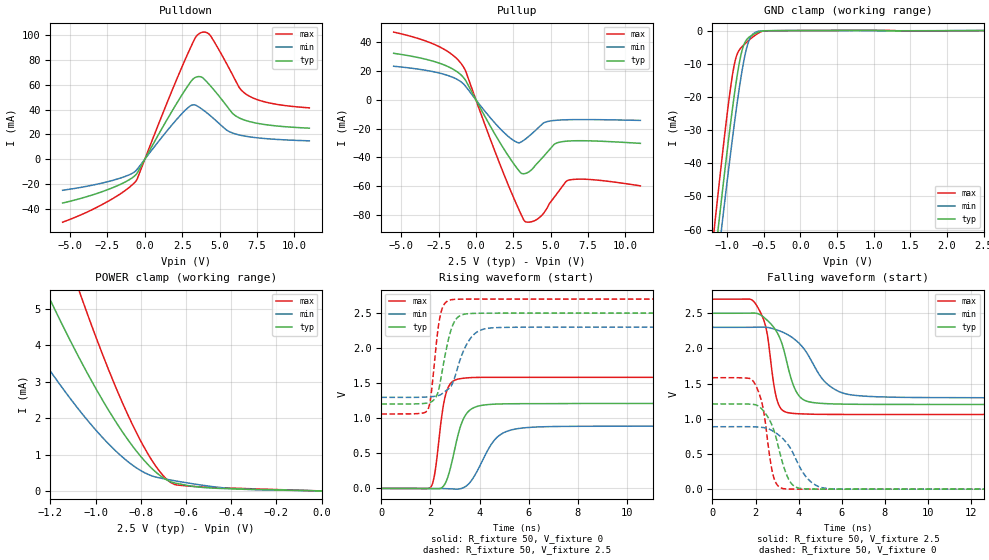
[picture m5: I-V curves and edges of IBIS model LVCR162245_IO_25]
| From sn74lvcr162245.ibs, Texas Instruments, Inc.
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[Model]   LVCR162245_IO_25
Model_type  I/O
Vinl=0.8
Vinh=2.0
Enable   Active-Low
Vref =   0
Rref =   500
Cref =   30p
Vmeas =   1.5
| variable   typ   min   max
C_comp   7.42pF   6.47pF   8.78pF
| C_pullup   5.98pF   4.73pF   8.31pF
| C_pulldown   5.48pF   4.75pF   6.82pF
| C_tri-state   7.42pF   6.47pF   8.78pF
[Temperature Range]   40   100   -40
| Ambient temperature   25   85   -40
[Voltage range]   2.5   2.3   2.7
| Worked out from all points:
|   slope of the pulldown table from 0 to 0.375 V, typ, clamps not added: 45.6 ohm
|   slope of the pullup table from 0 to 0.375 V, typ, clamps not added: 51.7 ohm
|   GND clamp passes 1 mA (typ) near -0.62 V on its own axis
|   POWER clamp passes 1 mA (typ) near -0.81 V on its own axis
|   rising waveform, R_fixture 50, V_fixture 0: 20-80 % time 538ps typ, 869ps min, 351ps max; typ from 0 V to 1.21 V
|   falling waveform, R_fixture 50, V_fixture 2.5: 20-80 % time 800ps typ, 1.38ns min, 491ps max; typ from 2.5 V to 1.2 V
|   rising waveform, R_fixture 50, V_fixture 2.5: 20-80 % time 451ps typ, 652ps min, 308ps max; typ from 1.2 V to 2.5 V
|   falling waveform, R_fixture 50, V_fixture 0: 20-80 % time 720ps typ, 1.04ns min, 472ps max; typ from 1.21 V to 0 V
[GND Clamp]
| LVCR162245_IO_25
|   Voltage   I(typ)   I(min)   I(max)
-5.5V     -1A        -986.6mA   -1.023A
-1.18V    -71.44mA   -79.99mA   -60.97mA
-1.13V    -61.52mA   -70.28mA   -50.73mA
-1.105V   -56.63mA   -65.48mA   -45.68mA
-1.08V    -51.77mA   -60.71mA   -40.71mA
-1.06V    -47.93mA   -56.93mA   -36.78mA
-965mV    -30.31mA   -39.41mA   -19.38mA
-885mV    -16.96mA   -25.59mA   -8.742mA
-810mV    -7.339mA   -14.11mA   -5.2mA
-745mV    -3.144mA   -6.398mA   -3.783mA
-625mV    -1.013mA   -674.6uA   -1.554mA
2.5V      57.27pA    21.9uA     -34.02uA
[POWER Clamp]
| LVCR162245_IO_25
|   Voltage   I(typ)   I(min)   I(max)
-5.5V     84.03mA    59.93mA    121.9mA
-1.42V    8.282mA    5.391mA    12.35mA
-1.215V   5.445mA    3.429mA    8.161mA
-1.19V    5.119mA    3.207mA    7.678mA
-1.085V   3.809mA    2.325mA    5.727mA
-1.06V    3.513mA    2.129mA    5.284mA
-945mV    2.246mA    1.311mA    3.375mA
-820mV    1.101mA    637.4uA    1.614mA
-735mV    526.2uA    383.5uA    693.8uA
-675mV    271.9uA    307.9uA    267.2uA
-385mV    56.11uA    57.39uA    74.69uA
-95.1fV   57.27pA    179.7pA    303pA
[Pulldown]
| LVCR162245_IO_25
|   Voltage   I(typ)   I(min)   I(max)
-5.5V     -35.33mA   -25.05mA   -50.76mA
-2.445V   -24.37mA   -18.03mA   -33.84mA
-595mV    -12.47mA   -9.27mA    -17.6mA
2.695V    55.75mA    39.35mA    80.16mA
3.22V     64.51mA    43.75mA    94.07mA
3.72V     66.37mA    41.15mA    101.7mA
4.385V    59.07mA    34.94mA    99.51mA
5.88V     36.75mA    21mA       67.58mA
6.33V     33.11mA    19.44mA    57.43mA
6.775V    31.04mA    18.39mA    52.29mA
8.31V     27.43mA    16.33mA    45.32mA
11V       24.96mA    14.76mA    41.31mA
[Pullup]
| LVCR162245_IO_25
|   Voltage   I(typ)   I(min)   I(max)
-5.5V     32.32mA    23.32mA    47.05mA
-2.535V   25.78mA    18.81mA    37.35mA
-1.57V    21.53mA    15.74mA    31.25mA
-920mV    16.54mA    11.89mA    24.26mA
-655mV    12.9mA     8.912mA    19.14mA
2.05V     -37.06mA   -24.39mA   -56.27mA
2.855V    -48.91mA   -29.86mA   -75.82mA
3.295V    -51.2mA    -27.42mA   -84.56mA
4.335V    -41.51mA   -17.84mA   -81.01mA
5.265V    -30.76mA   -14.32mA   -67.36mA
6.19V     -28.63mA   -13.83mA   -55.82mA
11V       -30.25mA   -14.3mA    -59.76mA
[Ramp]
| LVCR162245_IO_25
| variable   typ   min   max
dV/dt_r   0.73/5.45E-10   0.54/8.78E-10   0.95/3.54E-10
dV/dt_f   0.78/8.08E-10   0.60/1.39E-09   0.98/4.98E-10
R_load = 50
[Rising Waveform]
| LVCR162245_IO_25
R_fixture =   50
C_fixture =   0
L_fixture =   0
V_fixture =   0
V_fixture_min = 0
V_fixture_max = 0
|   Time   V(typ)   V(min)   V(max)
0s        407.6pV    1.25nV     4.231nV
2.03ns    -2.701mV   -1.091mV   26.79mV
2.19ns    -4.491mV   -1.437mV   242.7mV
2.46ns    10.29mV    -2.378mV   1.029V
2.615ns   80.92mV    -3.454mV   1.331V
3.185ns   840.8mV    -6.466mV   1.563V
3.8ns     1.157V     182.6mV    1.582V
4.675ns   1.203V     715.8mV    1.584V
5.71ns    1.208V     859.9mV    1.584V
24.99ns   1.211V     887.3mV    1.584V
[Falling Waveform]
| LVCR162245_IO_25
R_fixture =   50
C_fixture =   0
L_fixture =   0
V_fixture =   2.5
V_fixture_min = 2.3
V_fixture_max = 2.7
|   Time   V(typ)   V(min)   V(max)
0s        2.5V       2.3V       2.7V
2ns       2.502V     2.301V     2.635V
2.5ns     2.412V     2.301V     2.272V
3ns       2.227V     2.262V     1.265V
3.505ns   1.738V     2.193V     1.087V
3.835ns   1.419V     2.124V     1.075V
4.215ns   1.273V     2.007V     1.069V
5.255ns   1.216V     1.514V     1.062V
6.475ns   1.207V     1.338V     1.062V
24.99ns   1.204V     1.299V     1.062V
[Rising Waveform]
| LVCR162245_IO_25
R_fixture =   50
C_fixture =   0
L_fixture =   0
V_fixture =   2.5
V_fixture_min = 2.3
V_fixture_max = 2.7
|   Time   V(typ)   V(min)   V(max)
0s        1.204V     1.299V     1.062V
1.885ns   1.218V     1.304V     1.12V
2.01ns    1.23V      1.308V     1.292V
2.275ns   1.341V     1.32V      2.175V
2.405ns   1.527V     1.336V     2.473V
2.86ns    2.283V     1.469V     2.691V
3.135ns   2.447V     1.754V     2.698V
3.575ns   2.493V     2.112V     2.7V
4.41ns    2.499V     2.286V     2.7V
24.99ns   2.5V       2.3V       2.7V
[Falling Waveform]
| LVCR162245_IO_25
R_fixture =   50
C_fixture =   0
L_fixture =   0
V_fixture =   0
V_fixture_min = 0
V_fixture_max = 0
|   Time   V(typ)   V(min)   V(max)
0s        1.211V     887.3mV    1.584V
1.935ns   1.203V     886.1mV    1.516V
2.34ns    1.123V     876.7mV    1.167V
2.825ns   860.3mV    822.1mV    190.2mV
3.275ns   352.3mV    715.6mV    8.713mV
3.555ns   130.3mV    612.1mV    1.679mV
3.845ns   34.15mV    445mV      779.7uV
4.495ns   2.02mV     124.3mV    237.5uV
5.315ns   500.3uV    9.852mV    61.65uV
24.99ns   1.688uV    150.4nV    1.06uV
